| IBIS file stm32u3b5_3c5_ufbga132.ibs
[IBIS ver] 4.2
[File name] stm32u3b5_3c5_ufbga132.ibs
[File Rev] 0.1
[Date] 09-03-2026
[Source] Data Created at STMicroelectronics
[Notes]  File originated from ELDO simulations.
[Disclaimer]  This information is for modeling purpose only and is
   not guaranted. The information is subject to change without
   notice.
[Copyright] Copyright 2026 STMicroelectronics Inc.
|   Component stm32u3b5_3c5_ufbga132
[Component] stm32u3b5_3c5_ufbga132
[Manufacturer] STMicroelectronics
[Package]
| variable   typ   min   max
R_pkg  0  NA  NA
L_pkg  0  NA  NA
C_pkg  0  NA  NA
[Pin]   signal_name   model_name
A1  PE5  io8_ft_100m
A2  PE3  io8_ft_100m_hslv
A3  PE1  io8_ft_100m
A4  PB9  io8_ft_100m_hslv
A5  PB6  io8_ft_100m_hslv
A6  PG12  io8_ft_100m_hslv
A7  PD6  io8_ft_100m_hslv
A8  PD5  io8_ft_100m_hslv
A9  PD2  io8_ft_100m_hslv
A10  PC11  io8_ft_100m_hslv
A11  PA15  io8_ft_100m
A12  VDDUSB  power
B1  VBAT  power
B2  PE4  io8_ft_100m
B3  PE2  io8_ft_100m
B4  PG15  io8_ft_100m_hslv
B5  PH3-BOOT0  io8_ft_100m_hslv
B6  PB4  io8_ft_100m_hslv
B7  PG9  io8_ft_100m_hslv
B8  PD4  io8_ft_100m_hslv
B9  PD1  io8_ft_100m
B10  PC12  io8_ft_100m_hslv
B11  PC10  io8_ft_100m_hslv
B12  PA12  io8usb_ft_phy
C1  PC14-OSC32_IN  io_ft_tamp
C2  PE6  io8_ft_100m
C3  PC13  io8_ft_100m_v33
C4  PE0  io8_ft_100m
C5  PB8  io8_ft_100m_hslv
C6  PB3  io8_ft_100m_hslv
C7  PG10  io8_ft_100m_hslv
C8  PD3  io8_ft_100m_hslv
C9  PD0  io8_ft_100m
C10  PA13  io8_ft_100m
C11  PA14  io8_ft_100m
C12  PA11  io8usb_ft_phy
D1  PC15-OSC32_OUT  io_ft_tamp
D2  PF0  io8_ft_100m_hslv
D3  PF3  io8_ft_100m
D4  VDD  power
D5  PB7  io8_ft_100m_hslv
D6  PB5  io8_ft_100m_hslv
D7  PD7  io8_ft_100m_hslv
D8  VDDIO2  power
D9  VDD  power
D10  PA9  io8_ft_100m
D11  PA10  io8_ft_100m
D12  PA8  io8_ft_100m_hslv
E1  PF2  io8_ft_100m
E2  PF1  io8_ft_100m_hslv
E3  PF4  io8_ft_100m
E4  VSS  gnd
E9  VSS  gnd
E10  PC7  io8_ft_100m_hslv
E11  PC9  io8_ft_100m_hslv
E12  PC8  io8_ft_100m_hslv
F1  PH0-OSC_IN  io8_ft_100m
F2  PF5  io8_ft_100m
F3  PC2  io8_ft_100m_hslv
F4  PC3  io8_ft_100m_hslv
F6  VSS  gnd
F7  VDD  power
F9  PG6  io8_ft_100m_hslv
F10  PG7  io8_ft_100m_hslv
F11  PC6  io8_ft_100m_hslv
F12  PG8  io8_ft_100m_hslv
G1  PH1-OSC_OUT  io8_ft_100m
G2  NRST  ioreset_v33
G3  PC1  io8_ft_100m_hslv
G4  PA1  io8_ft_100m_hslv
G6  VDD  power
G7  VSS  gnd
G9  PG4  io8_ft_100m_hslv
G10  PG2  io8_ft_100m_hslv
G11  PG3  io8_ft_100m_hslv
G12  PG5  io8_ft_100m_hslv
H1  VSSA_VREFM  nc
H2  PC0  io8_ft_100m_hslv
H3  OPAMP1_VINM  io8_ft_100m_hslv
H4  VSS  gnd
H9  VSS  gnd
H10  PD14  io8_ft_100m
H11  PD13  io8_ft_100m_hslv
H12  PD15  io8_ft_100m
J1  VREFP  nc
J2  PA0  io8_ft_100m
J3  PC5  io8_ft_100m
J4  VDD  power
J5  PF14  io8_ft_100m_hslv
J6  PE8  io8_ft_100m
J7  PE10  io8_ft_100m_hslv
J8  PE12  io8_ft_100m_hslv
J9  VDD  power
J10  PD9  io8_ft_100m
J11  PD11  io8_ft_100m_hslv
J12  PD12  io8_ft_100m_hslv
K1  VDDA  nc
K2  PA2  io8_ft_100m_hslv
K3  PA7  io8_ft_100m_hslv
K4  PB2  io8_ft_100m_hslv
K5  PF11  io8_ft_100m_hslv
K6  PG1  io8_ft_100m
K7  PE7  io8_ft_100m
K8  PE14  io8_ft_100m_hslv
K9  PB10  io8_ft_100m_hslv
K10  PB13  io8_ft_100m_hslv
K11  PB14  io8_ft_100m_hslv
K12  PB15  io8_ft_100m
L1  PA3  io8_ft_100m_hslv
L2  PA6  io8_ft_100m_hslv
L3  PA4  io8_ft_100m_hslv
L4  PB1  io8_ft_100m_hslv
L5  PF12  io8_ft_100m
L6  PF15  io8_ft_100m_hslv
L7  PE11  io8_ft_100m_hslv
L8  PE15  io8_ft_100m_hslv
L9  PB11  io8_ft_100m_hslv
L10  VCAP  nc
L11  PB12  io8_ft_100m_hslv
L12  PD8  io8_ft_100m
M1  PA5  io8_ft_100m
M2  OPAMP2_VINM  io8_ft_100m_hslv
M3  PC4  io8_ft_100m_hslv
M4  PB0  io8_ft_100m_hslv
M5  PF13  io8_ft_100m
M6  PG0  io8_ft_100m
M7  PE9  io8_ft_100m_hslv
M8  PE13  io8_ft_100m_hslv
M9  PG14  io8_ft_100m_hslv
M10  PG13  io8_ft_100m_hslv
M11  PG11  io8_ft_100m_hslv
M12  PD10  io8_ft_100m
[Package Model]   42a-ufbga-7x7-132-ldo-260213
[Pin Mapping]   pulldown_ref   pullup_ref   | Comment
A1  gndio  vddio
A2  gndio  vddio
A3  gndio  vddio
A4  gndio  vddio
A5  gndio  vddio
A6  gndio  vddio2
A7  gndio  vddio
A8  gndio  vddio
A9  gndio  vddio
A10  gndio  vddio
A11  gndio  vddio
A12  nc  vddusb
B1  nc  vsw
B2  gndio  vddio
B3  gndio  vddio
B4  gndio  vddio2
B5  gndio  vddio
B6  gndio  vddio
B7  gndio  vddio2
B8  gndio  vddio
B9  gndio  vddio
B10  gndio  vddio
B11  gndio  vddio
B12  gndio  vddusb  | Depending on IO usage
| B12  gndio  vddio  | Depending on IO usage
C1  gndio  vsw
C2  gndio  vddio
C3  gndio  vsw
C4  gndio  vddio
C5  gndio  vddio
C6  gndio  vddio
C7  gndio  vddio2
C8  gndio  vddio
C9  gndio  vddio
C10  gndio  vddio
C11  gndio  vddio
C12  gndio  vddusb  | Depending on IO usage
| C12  gndio  vddio  | Depending on IO usage
D1  gndio  vsw
D2  gndio  vddio
D3  gndio  vddio
D4  nc  vddio
D5  gndio  vddio
D6  gndio  vddio
D7  gndio  vddio
D8  nc  vddio2
D9  nc  vddio
D10  gndio  vddio
D11  gndio  vddio
D12  gndio  vddio
E1  gndio  vddio
E2  gndio  vddio
E3  gndio  vddio
E4  gndio  nc
E9  gndio  nc
E10  gndio  vddio
E11  gndio  vddio
E12  gndio  vddio
F1  gndio  vddio
F2  gndio  vddio
F3  gndio  vddio
F4  gndio  vddio
F6  gndio  nc
F7  nc  vddio
F9  gndio  vddio2
F10  gndio  vddio2
F11  gndio  vddio
F12  gndio  vddio2
G1  gndio  vddio
G2  gndio  vddio
G3  gndio  vddio
G4  gndio  vddio
G6  nc  vddio
G7  gndio  nc
G9  gndio  vddio2
G10  gndio  vddio2
G11  gndio  vddio2
G12  gndio  vddio2
H1  nc  nc
H2  gndio  vddio
H3  gndio  vddio
H4  gndio  nc
H9  gndio  nc
H10  gndio  vddio
H11  gndio  vddio
H12  gndio  vddio
J1  nc  nc
J2  gndio  vddio
J3  gndio  vddio
J4  nc  vddio
J5  gndio  vddio
J6  gndio  vddio
J7  gndio  vddio
J8  gndio  vddio
J9  nc  vddio
J10  gndio  vddio
J11  gndio  vddio
J12  gndio  vddio
K1  nc  nc
K2  gndio  vddio
K3  gndio  vddio
K4  gndio  vddio
K5  gndio  vddio
K6  gndio  vddio
K7  gndio  vddio
K8  gndio  vddio
K9  gndio  vddio
K10  gndio  vddio
K11  gndio  vddio
K12  gndio  vddio
L1  gndio  vddio
L2  gndio  vddio
L3  gndio  vddio
L4  gndio  vddio
L5  gndio  vddio
L6  gndio  vddio
L7  gndio  vddio
L8  gndio  vddio
L9  gndio  vddio
L10  nc  nc
L11  gndio  vddio
L12  gndio  vddio
M1  gndio  vddio
M2  gndio  vddio
M3  gndio  vddio
M4  gndio  vddio
M5  gndio  vddio
M6  gndio  vddio
M7  gndio  vddio
M8  gndio  vddio
M9  gndio  vddio2
M10  gndio  vddio2
M11  gndio  vddio2
M12  gndio  vddio
|[Diff Pin]  inv_pin  vdiff  tdelay_typ  tdelay_min  tdelay_max
|B12  C12  NA  NA  NA  NA
[Model Selector] io8_ft_100m
io8_ft_100m_ls_1v2  "GPIO 100MHz - 5V tolerant - low speed - 1.2V range"
io8_ft_100m_ls_1v8  "GPIO 100MHz - 5V tolerant - low speed - 1.8V range"
io8_ft_100m_ls_3v3  "GPIO 100MHz - 5V tolerant - low speed - 3.3V range"
io8_ft_100m_ms_1v2  "GPIO 100MHz - 5V tolerant - med speed - 1.2V range"
io8_ft_100m_ms_1v8  "GPIO 100MHz - 5V tolerant - med speed - 1.8V range"
io8_ft_100m_ms_3v3  "GPIO 100MHz - 5V tolerant - med speed - 3.3V range"
io8_ft_100m_fs_1v2  "GPIO 100MHz - 5V tolerant - fast speed - 1.2V range"
io8_ft_100m_fs_1v8  "GPIO 100MHz - 5V tolerant - fast speed - 1.8V range"
io8_ft_100m_fs_3v3  "GPIO 100MHz - 5V tolerant - fast speed - 3.3V range"
io8_ft_100m_hs_1v2  "GPIO 100MHz - 5V tolerant - high speed - 1.2V range"
io8_ft_100m_hs_1v8  "GPIO 100MHz - 5V tolerant - high speed - 1.8V range"
io8_ft_100m_hs_3v3  "GPIO 100MHz - 5V tolerant - high speed - 3.3V range"
[Model Selector] io8_ft_100m_hslv
io8_ft_100m_ls_1v2  "GPIO 100MHz - 5V tolerant - low speed - 1.2V range"
io8_ft_100m_ls_1v8  "GPIO 100MHz - 5V tolerant - low speed - 1.8V range"
io8_ft_100m_ls_3v3  "GPIO 100MHz - 5V tolerant - low speed - 3.3V range"
io8_ft_100m_ms_1v2  "GPIO 100MHz - 5V tolerant - med speed - 1.2V range"
io8_ft_100m_ms_1v8  "GPIO 100MHz - 5V tolerant - med speed - 1.8V range"
io8_ft_100m_ms_3v3  "GPIO 100MHz - 5V tolerant - med speed - 3.3V range"
io8_ft_100m_fs_1v2  "GPIO 100MHz - 5V tolerant - fast speed - 1.2V range"
io8_ft_100m_fs_1v8  "GPIO 100MHz - 5V tolerant - fast speed - 1.8V range"
io8_ft_100m_fs_3v3  "GPIO 100MHz - 5V tolerant - fast speed - 3.3V range"
io8_ft_100m_hs_1v2  "GPIO 100MHz - 5V tolerant - high speed - 1.2V range"
io8_ft_100m_hs_1v8  "GPIO 100MHz - 5V tolerant - high speed - 1.8V range"
io8_ft_100m_hs_3v3  "GPIO 100MHz - 5V tolerant - high speed - 3.3V range"
io8_ft_100m_hslv_ls_1v2  "GPIO 100MHz low voltage optimization - 5V tolerant - low speed - 1.2V range"
io8_ft_100m_hslv_ls_1v8  "GPIO 100MHz low voltage optimization - 5V tolerant - low speed - 1.8V range"
io8_ft_100m_hslv_ls_2v5  "GPIO 100MHz low voltage optimization - 5V tolerant - low speed - 3.3V range"
io8_ft_100m_hslv_ms_1v2  "GPIO 100MHz low voltage optimization - 5V tolerant - med speed - 1.2V range"
io8_ft_100m_hslv_ms_1v8  "GPIO 100MHz low voltage optimization - 5V tolerant - med speed - 1.8V range"
io8_ft_100m_hslv_ms_2v5  "GPIO 100MHz low voltage optimization - 5V tolerant - med speed - 3.3V range"
io8_ft_100m_hslv_fs_1v2  "GPIO 100MHz low voltage optimization - 5V tolerant - fast speed - 1.2V range"
io8_ft_100m_hslv_fs_1v8  "GPIO 100MHz low voltage optimization - 5V tolerant - fast speed - 1.8V range"
io8_ft_100m_hslv_fs_2v5  "GPIO 100MHz low voltage optimization - 5V tolerant - fast speed - 3.3V range"
io8_ft_100m_hslv_hs_1v2  "GPIO 100MHz low voltage optimization - 5V tolerant - high speed - 1.2V range"
io8_ft_100m_hslv_hs_1v8  "GPIO 100MHz low voltage optimization - 5V tolerant - high speed - 1.8V range"
io8_ft_100m_hslv_hs_2v5  "GPIO 100MHz low voltage optimization - 5V tolerant - high speed - 3.3V range"
[Model Selector] io8_ft_100m_v33
io8_ft_100m_v33_ls_1v2  "GPIO_V33 100MHz - 5V tolerant - low speed - 1.2V range"
io8_ft_100m_v33_ls_1v8  "GPIO_V33 100MHz - 5V tolerant - low speed - 1.8V range"
io8_ft_100m_v33_ls_3v3  "GPIO_V33 100MHz - 5V tolerant - low speed - 3.3V range"
io8_ft_100m_v33_ms_1v2  "GPIO_V33 100MHz - 5V tolerant - med speed - 1.2V range"
io8_ft_100m_v33_ms_1v8  "GPIO_V33 100MHz - 5V tolerant - med speed - 1.8V range"
io8_ft_100m_v33_ms_3v3  "GPIO_V33 100MHz - 5V tolerant - med speed - 3.3V range"
io8_ft_100m_v33_fs_1v2  "GPIO_V33 100MHz - 5V tolerant - fast speed - 1.2V range"
io8_ft_100m_v33_fs_1v8  "GPIO_V33 100MHz - 5V tolerant - fast speed - 1.8V range"
io8_ft_100m_v33_fs_3v3  "GPIO_V33 100MHz - 5V tolerant - fast speed - 3.3V range"
io8_ft_100m_v33_hs_1v2  "GPIO_V33 100MHz - 5V tolerant - high speed - 1.2V range"
io8_ft_100m_v33_hs_1v8  "GPIO_V33 100MHz - 5V tolerant - high speed - 1.8V range"
io8_ft_100m_v33_hs_3v3  "GPIO_V33 100MHz - 5V tolerant - high speed - 3.3V range"
[Model Selector] io8usb_ft_phy
io8_ft_100m_ls_1v2  "GPIO 100MHz - 5V tolerant - low speed - 1.2V range"
io8_ft_100m_ls_1v8  "GPIO 100MHz - 5V tolerant - low speed - 1.8V range"
io8_ft_100m_ls_3v3  "GPIO 100MHz - 5V tolerant - low speed - 3.3V range"
io8_ft_100m_ms_1v2  "GPIO 100MHz - 5V tolerant - med speed - 1.2V range"
io8_ft_100m_ms_1v8  "GPIO 100MHz - 5V tolerant - med speed - 1.8V range"
io8_ft_100m_ms_3v3  "GPIO 100MHz - 5V tolerant - med speed - 3.3V range"
io8_ft_100m_fs_1v2  "GPIO 100MHz - 5V tolerant - fast speed - 1.2V range"
io8_ft_100m_fs_1v8  "GPIO 100MHz - 5V tolerant - fast speed - 1.8V range"
io8_ft_100m_fs_3v3  "GPIO 100MHz - 5V tolerant - fast speed - 3.3V range"
io8_ft_100m_hs_1v2  "GPIO 100MHz - 5V tolerant - high speed - 1.2V range"
io8_ft_100m_hs_1v8  "GPIO 100MHz - 5V tolerant - high speed - 1.8V range"
io8_ft_100m_hs_3v3  "GPIO 100MHz - 5V tolerant - high speed - 3.3V range"
io8usb_ft_phy_hs_3v3   "USB full speed"
io8usb_ft_phy_ls_3v3   "USB low speed"
[Model Selector] io_ft_tamp
io_ft_tamp_ls_1v2 "io8_ft tamp low speed @ 1.2V"
io_ft_tamp_ls_1v8 "io8_ft tamp low speed @ 1.8V"
io_ft_tamp_ls_3v3 "io8_ft tamp low speed @ 3.3V"
io_ft_tamp_ms_1v2 "io8_ft tamp med speed @ 1.2V"
io_ft_tamp_ms_1v8 "io8_ft tamp med speed @ 1.8V"
io_ft_tamp_ms_3v3 "io8_ft tamp med speed @ 3.3V"
io_ft_tamp_fs_1v2 "io8_ft tamp fast speed @ 1.2V"
io_ft_tamp_fs_1v8 "io8_ft tamp fast speed @ 1.8V"
io_ft_tamp_fs_3v3 "io8_ft tamp fast speed @ 3.3V"
io_ft_tamp_hs_1v2 "io8_ft tamp high speed @ 1.2V"
io_ft_tamp_hs_1v8 "io8_ft tamp high speed @ 1.8V"
io_ft_tamp_hs_3v3 "io8_ft tamp high speed @ 3.3V"
[Model Selector] ioreset_v33
ioreset_v33_1v2 "Reset PAD. 5V tolerant. 1.2V range"
ioreset_v33_1v8 "Reset PAD. 5V tolerant. 1.8V range"
ioreset_v33_3v3 "Reset PAD. 5V tolerant. 3.3V range"
[Define Package Model]  42a-ufbga-7x7-132-ldo-260213
[Manufacturer]  unknown
[OEM]  unknown
[Description]  unknown
[Number Of Pins]  122
[Pin Numbers]
| Pin Name Terminal   Net Name   Starting Node   Ending Node
G2 | NRST
J2 | PA0
G4 | PA1
H3 | OPAMP1_VINM
K2 | PA2
L1 | PA3
L3 | PA4
M1 | PA5
L2 | PA6
K3 | PA7
M2 | OPAMP2_VINM
D12 | PA8
D10 | PA9
D11 | PA10
C12 | PA11
B12 | PA12
C10 | PA13
C11 | PA14
A11 | PA15
M4 | PB0
L4 | PB1
K4 | PB2
C6 | PB3
B6 | PB4
D6 | PB5
A5 | PB6
D5 | PB7
C5 | PB8
A4 | PB9
K9 | PB10
L9 | PB11
L11 | PB12
K10 | PB13
K11 | PB14
K12 | PB15
H2 | PC0
G3 | PC1
F3 | PC2
F4 | PC3
M3 | PC4
J3 | PC5
F11 | PC6
E10 | PC7
E12 | PC8
E11 | PC9
B11 | PC10
A10 | PC11
B10 | PC12
C3 | PC13
C1 | PC14-OSC32_IN
D1 | PC15-OSC32_OUT
C9 | PD0
B9 | PD1
A9 | PD2
C8 | PD3
B8 | PD4
A8 | PD5
A7 | PD6
D7 | PD7
L12 | PD8
J10 | PD9
M12 | PD10
J11 | PD11
J12 | PD12
H11 | PD13
H10 | PD14
H12 | PD15
C4 | PE0
A3 | PE1
B3 | PE2
A2 | PE3
B2 | PE4
A1 | PE5
C2 | PE6
K7 | PE7
J6 | PE8
M7 | PE9
J7 | PE10
L7 | PE11
J8 | PE12
M8 | PE13
K8 | PE14
L8 | PE15
D2 | PF0
E2 | PF1
E1 | PF2
D3 | PF3
E3 | PF4
F2 | PF5
K5 | PF11
L5 | PF12
M5 | PF13
J5 | PF14
L6 | PF15
M6 | PG0
K6 | PG1
G10 | PG2
G11 | PG3
G9 | PG4
G12 | PG5
F9 | PG6
F10 | PG7
F12 | PG8
B7 | PG9
C7 | PG10
M11 | PG11
A6 | PG12
M10 | PG13
M9 | PG14
B4 | PG15
F1 | PH0-OSC_IN
G1 | PH1-OSC_OUT
B5 | PH3-BOOT0
B1 | VBAT
L10 | VCAP
D4 | VDD
K1 | VDDA
D8 | VDDIO2
A12 | VDDUSB
J1 | VREFP
E4 | VSS
H1 | VSSA_VREFM
|[Merged Pins]  D4
|D9  |  VDD
|F7  |  VDD
|G6  |  VDD
|J4  |  VDD
|J9  |  VDD
|[Merged Pins]  E4
|E9  |  VSS
|F6  |  VSS
|G7  |  VSS
|H4  |  VSS
|H9  |  VSS
[Model Data]
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[End Model Data]
[End Package Model]
|End [Component]
| Models and submodels in the file (53): io8_ft_100m_fs_1v2 (I/O), io8_ft_100m_fs_1v8 (I/O), io8_ft_100m_fs_3v3 (I/O), io8_ft_100m_hs_1v2 (I/O), io8_ft_100m_hs_1v8 (I/O), io8_ft_100m_hs_3v3 (I/O), io8_ft_100m_hslv_fs_1v2 (I/O), io8_ft_100m_hslv_fs_1v8 (I/O), io8_ft_100m_hslv_fs_2v5 (I/O), io8_ft_100m_hslv_hs_1v2 (I/O), io8_ft_100m_hslv_hs_1v8 (I/O), io8_ft_100m_hslv_hs_2v5 (I/O), io8_ft_100m_hslv_ls_1v2 (I/O), io8_ft_100m_hslv_ls_1v8 (I/O), io8_ft_100m_hslv_ls_2v5 (I/O), io8_ft_100m_hslv_ms_1v2 (I/O), io8_ft_100m_hslv_ms_1v8 (I/O), io8_ft_100m_hslv_ms_2v5 (I/O), io8_ft_100m_ls_1v2 (I/O), io8_ft_100m_ls_1v8 (I/O), io8_ft_100m_ls_3v3 (I/O), io8_ft_100m_ms_1v2 (I/O), io8_ft_100m_ms_1v8 (I/O), io8_ft_100m_ms_3v3 (I/O), io8_ft_100m_v33_fs_1v2 (I/O), io8_ft_100m_v33_fs_1v8 (I/O), io8_ft_100m_v33_fs_3v3 (I/O), io8_ft_100m_v33_hs_1v2 (I/O), io8_ft_100m_v33_hs_1v8 (I/O), io8_ft_100m_v33_hs_3v3 (I/O), io8_ft_100m_v33_ls_1v2 (I/O), io8_ft_100m_v33_ls_1v8 (I/O), io8_ft_100m_v33_ls_3v3 (I/O), io8_ft_100m_v33_ms_1v2 (I/O), io8_ft_100m_v33_ms_1v8 (I/O), io8_ft_100m_v33_ms_3v3 (I/O), io8usb_ft_phy_hs_3v3 (I/O), io8usb_ft_phy_ls_3v3 (I/O), io_ft_tamp_fs_1v2 (I/O), io_ft_tamp_fs_1v8 (I/O), io_ft_tamp_fs_3v3 (I/O), io_ft_tamp_hs_1v2 (I/O), io_ft_tamp_hs_1v8 (I/O), io_ft_tamp_hs_3v3 (I/O), io_ft_tamp_ls_1v2 (I/O), io_ft_tamp_ls_1v8 (I/O), io_ft_tamp_ls_3v3 (I/O), io_ft_tamp_ms_1v2 (I/O), io_ft_tamp_ms_1v8 (I/O), io_ft_tamp_ms_3v3 (I/O), ioreset_v33_1v2 (I/O_open_drain), ioreset_v33_1v8 (I/O_open_drain), ioreset_v33_3v3 (I/O_open_drain)
